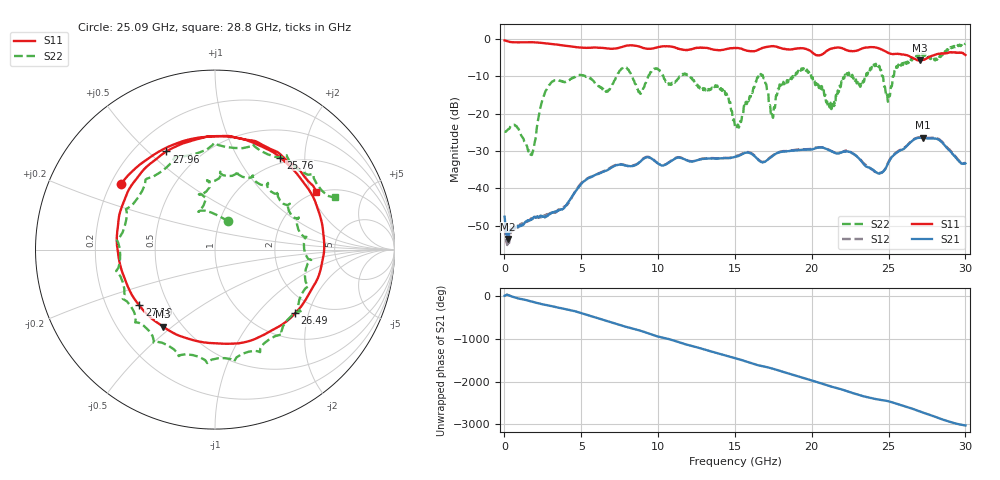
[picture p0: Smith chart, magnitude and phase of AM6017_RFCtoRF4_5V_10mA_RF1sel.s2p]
!Agilent Technologies,E8364B,MY43040894,A.07.50.67
!Agilent E8364B: A.07.50.67
!Date: Tuesday, August 21, 2018 13:29:59
!Correction: S11(Full 2 Port(1,2))
!S21(Full 2 Port(1,2))
!S12(Full 2 Port(1,2))
!S22(Full 2 Port(1,2))
!S2P File: Measurements: S11, S21, S12, S22:
# Hz S  dB  R 50
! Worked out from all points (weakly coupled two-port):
!   1601 points, 10 MHz to 30 GHz, reference 50 ohm
!   highest |S21| = -26.40 dB at 27.23 GHz (marker M1); lowest = -53.6 dB at 234.9 MHz (marker M2)
!   lowest |S11| = -5.7 dB at 27.06 GHz (marker M3), VSWR 3.15, Z = 19.9 - j23.3 ohm
!   |S11| at or under -10 dB: nowhere
!   |S22| runs from -31.1 to -1.2 dB; largest |S21 - S12| = 0.0022
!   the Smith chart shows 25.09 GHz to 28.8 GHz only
!   S11 on the Smith chart (normalised r, x): 25.09 GHz: 0.24, +0.30; 25.76 GHz: 0.91, +1.54; 26.49 GHz: 1.56, -1.64; 27.19 GHz: 0.34, -0.29; 27.96 GHz: 0.33, +0.57; 28.8 GHz: 1.97, +2.19
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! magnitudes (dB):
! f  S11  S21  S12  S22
! 10 MHz  -0.4  -47.6  -50.3  -24.8
! 234.9 MHz  -0.7  -53.6  -55.5  -24.2
! 1.772 GHz  -0.8  -48.3  -48.0  -31.1
! 2.803 GHz  -1.2  -47.3  -46.9  -13.0
! 5.015 GHz  -2.3  -38.8  -38.5  -9.6
! 10.02 GHz  -2.1  -33.4  -33.4  -8.2
! 15.01 GHz  -2.4  -31.6  -31.4  -23.4
! 16.58 GHz  -2.8  -32.6  -32.5  -9.6
! 17.46 GHz  -1.9  -31.3  -31.2  -20.9
! 20.01 GHz  -3.5  -29.6  -29.4  -10.5
! 21.28 GHz  -2.5  -30.1  -30.0  -18.8
! 24.19 GHz  -2.3  -35.7  -35.8  -6.9
! 25.01 GHz  -3.7  -33.0  -32.7  -15.0
! 25.09 GHz  -3.9  -32.4  -32.2  -15.2
! 25.76 GHz  -4.0  -29.9  -29.7  -6.7
! 26.49 GHz  -4.9  -27.4  -27.3  -5.6
! 27.06 GHz  -5.7  -26.4  -26.4  -4.0
! 27.19 GHz  -5.6  -26.4  -26.3  -4.2
! 27.23 GHz  -5.6  -26.4  -26.3  -4.4
! 27.96 GHz  -4.3  -26.6  -26.5  -5.5
! 28.8 GHz  -3.7  -29.2  -29.0  -2.7
! 30 GHz  -4.3  -33.3  -33.2  -1.2
